FUNCTION_BLOCK EL1008
VAR
	Channels : ARRAY [0..7] OF DigitalInputChannel;
END_VAR

METHOD PUBLIC GetDigitalInput : I_DigitalInput
VAR_INPUT
	channelNumber : INT;
END_VAR
GetDigitalInput := Channels[channelNumber];
END_METHOD

END_FUNCTION_BLOCK
